TYPE ST_DrvIn :
STRUCT
	Limit_Neg:BOOL;(*正限位*)
	Limit_Pos:BOOL;(*负限位*)
	HomeSensor:BOOL;(*原点开关*)

	Drive_Alarm:BOOL;(*驱动器报警*)
	Drive_Ready:BOOL;(*驱动器准备好*)
	Drive_Torque:DINT;(*1000对应100%额定转矩*)
	DC_Voltage:UDINT;(*驱动器直流母线电压*)
END_STRUCT
END_TYPE
